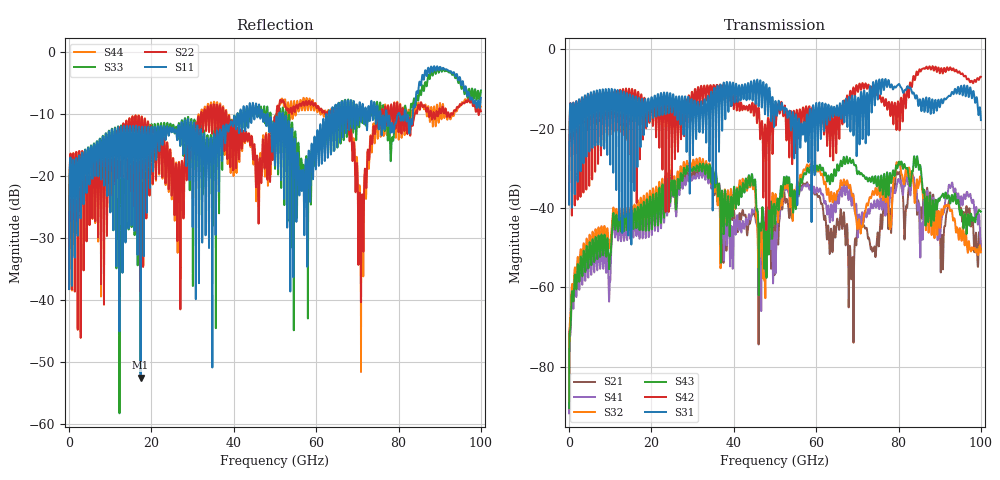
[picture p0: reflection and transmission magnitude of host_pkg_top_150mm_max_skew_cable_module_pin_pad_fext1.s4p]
# Hz S RI R 50
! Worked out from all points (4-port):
!   10000 points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, 10 MHz to 100 GHz, reference 50 ohm
!   strongest paths, dB at 10 MHz, 25.01 GHz, 50.01 GHz, 75.01 GHz, 100 GHz:
!     S31: -39.1, -14.7, -14.0, -12.2, -17.9
!     S42: -39.1, -23.6, -16.0, -11.7, -6.9
!     S43: -90.4, -32.2, -43.6, -32.3, -40.9
!     S32: -88.7, -31.7, -38.9, -35.5, -51.1
!     S41: -91.7, -33.6, -47.1, -38.6, -49.6
!     S21: -89.7, -33.0, -46.0, -46.7, -50.4
!   lowest |S11| = -52.6 dB at 17.37 GHz (marker M1), VSWR 1.00, Z = 50 + j0.231 ohm
!   |S11| at or under -10 dB: start of sweep to 40.88 GHz; 48.2 GHz to 51.06 GHz (2.856 GHz wide, 5.76 % of centre); 51.9 GHz to 63.12 GHz (11.22 GHz wide, 19.5 % of centre)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
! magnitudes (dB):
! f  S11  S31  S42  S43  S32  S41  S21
! 10 MHz  -38.3  -39.1  -39.1  -90.4  -88.7  -91.7  -89.7
! 17.37 GHz  -52.6  -23.1  -12.9  -39.3  -37.4  -41.7  -39.5
! 47.4 GHz  -10.1  -11.4  -22.4  -53.6  -57.4  -46.0  -47.7
! 57.99 GHz  -20.3  -20.4  -17.4  -30.0  -29.5  -34.0  -34.2
! 68.79 GHz  -12.1  -12.0  -11.6  -28.1  -37.0  -37.9  -52.4
! 79.92 GHz  -10.0  -8.9  -13.3  -28.9  -29.1  -32.7  -31.3
! 100 GHz  -7.5  -17.9  -6.9  -40.9  -51.1  -49.6  -50.4
